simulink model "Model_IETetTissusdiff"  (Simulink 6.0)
settings: Solver=ode45  StartTime=0.0  StopTime=16*t0  RelTol=1e-3
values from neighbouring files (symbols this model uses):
  beta = 0.95    [Constantes.m]    (also in ConstantesBck.m; ResCourV1.m = 1; ResCrV1.m = 1; ResEnerV1.m = 1)
  C = 1    [Constantes.m]    (also in ConstantesBck.m)
  Cdl = 603E-9    (= 6.03e-07)    [Constantes.m]    (also in ConstantesBck.m; ResCourV1.m = 7.313e-07; ResCrV1.m = 7.313e-07; ResEnerV1.m = 7.313e-07)
  const = 1E4    (= 10000)    [ConstantesBck.m]
  Fact = 10^2    (= 100)    [Constantes.m]    (also in ConstantesBck.m)
  gk = 36    [Constantes.m]    (also in ConstantesBck.m; sim_hh.m)
  gl = 0.3    [Constantes.m]    (also in ConstantesBck.m; sim_hh.m)
  gna = 120    [Constantes.m]    (also in ConstantesBck.m; sim_hh.m)
  h0 = 0.5961    [Constantes.m]    (also in ConstantesBck.m)
  Istim = 200E-6    (= 0.0002)    [Constantes.m]    (also in ConstantesBck.m = 5e-05)
  k = vth/pot    [CalculCharge.m]
  m0 = 0.0529    [Constantes.m]    (also in ConstantesBck.m)
  n0 = 0.3177    [Constantes.m]    (also in ConstantesBck.m)
  Rct = 185.6E3    (= 185600)    [Constantes.m]    (also in ConstantesBck.m; ResCourV1.m = 605200; ResCrV1.m = 605200; ResEnerV1.m = 605200)
  Rext = 2.9E3    (= 2900)    [Constantes.m]    (also in ConstantesBck.m)
  Rint = 2.9E2    (= 290)    [Constantes.m]    (also in ConstantesBck.m = 400)
  S = 3.14E-3    (= 0.00314)    [Constantes.m]    (also in ConstantesBck.m = 3.14e-09; ImpedanceZtissus.m = 4e-06; Ztissus.m = 4e-06)
  sigma = 66466    [Constantes.m]    (also in ConstantesBck.m; ResCourV1.m = 68000; ResCrV1.m = 68000; ResEnerV1.m = 68000)
  t0 = 2E-3    (= 0.002)    [Constantes.m]    (also in ConstantesBck.m = 0.001)
  Vdd = 3.3*Rcan/Rct*1000    (= 3.2147881681)    [Constantes.m]    (also in ConstantesBck.m = 1.8)
  Vk = -82    [Constantes.m]    (also in ConstantesBck.m)
  Vl = -59    [Constantes.m]    (also in ConstantesBck.m)
  Vna = 45    [Constantes.m]    (also in ConstantesBck.m)

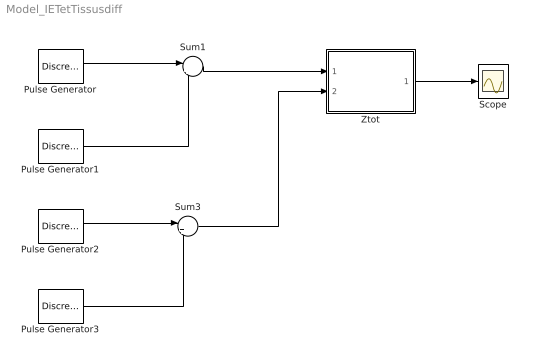
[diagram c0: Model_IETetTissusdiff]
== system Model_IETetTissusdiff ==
  Pulse Generator : DiscretePulseGenerator  PulseType=Time based  Amplitude=-Istim  Period=t0  PulseWidth=50
  Pulse Generator1 : DiscretePulseGenerator  PulseType=Time based  Amplitude=Istim  Period=t0  PulseWidth=50  PhaseDelay=t0/2
  Pulse Generator2 : DiscretePulseGenerator  PulseType=Time based  Amplitude=Vdd/2  Period=t0  PulseWidth=50
  Pulse Generator3 : DiscretePulseGenerator  PulseType=Time based  Amplitude=-Vdd/2  Period=t0  PulseWidth=50  PhaseDelay=t0/2
  Scope : Scope
  Sum1 : Sum  Inputs=|++
  Sum3 : Sum  Inputs=|++
  Ztot : Subsystem
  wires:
  Pulse Generator/1 -> Sum1/1
  Pulse Generator1/1 -> Sum1/2
  Sum1/1 -> Ztot/1(InZtot)
  Pulse Generator2/1 -> Sum3/1
  Pulse Generator3/1 -> Sum3/2
  Ztot/1(OutZtot) -> Scope/1
  Sum3/1 -> Ztot/2(InVRef)

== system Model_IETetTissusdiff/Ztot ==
  InZtot : Inport  Port=1  LatchInput=off
  InVRef : Inport  Port=2  LatchInput=off
  Gain : Gain
  Sum : Sum  Inputs=|++
  ZTissus : Subsystem
  Ziet : Subsystem
  OutZtot : Outport
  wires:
  Ziet/1(OutZiet) -> Gain/1
  InZtot/1 -> Ziet/1(InZiet), ZTissus/1(IStim)
  Gain/1 -> Sum/2
  Sum/1 -> OutZtot/1
  InVRef/1 -> ZTissus/2(Vref)
  ZTissus/1(Vout) -> Sum/1

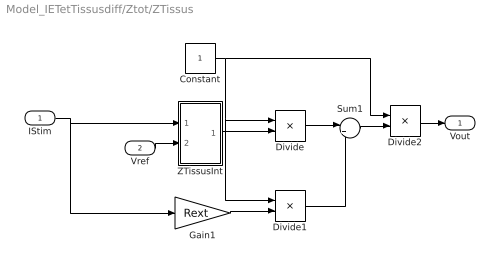
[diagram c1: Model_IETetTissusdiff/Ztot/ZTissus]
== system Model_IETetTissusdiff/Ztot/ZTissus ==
  IStim : Inport  Port=1  LatchInput=off
  Vref : Inport  Port=2  LatchInput=off
  Constant : Constant
  Divide : Product  Inputs=*/  OutScaling=2^-10
  Divide1 : Product  Inputs=*/  OutScaling=2^-10
  Divide2 : Product  Inputs=*/  OutScaling=2^-10
  Gain1 : Gain  Gain=Rext
  Sum1 : Sum  Inputs=|++
  ZTissusInt : Subsystem
  Vout : Outport
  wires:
  IStim/1 -> ZTissusInt/1(InStim), Gain1/1
  Constant/1 -> Divide/1, Divide1/1, Divide2/1
  ZTissusInt/1(Vout) -> Divide/2
  Gain1/1 -> Divide1/2
  Divide/1 -> Sum1/1
  Divide1/1 -> Sum1/2
  Sum1/1 -> Divide2/2
  Divide2/1 -> Vout/1
  Vref/1 -> ZTissusInt/2(VRefIn)

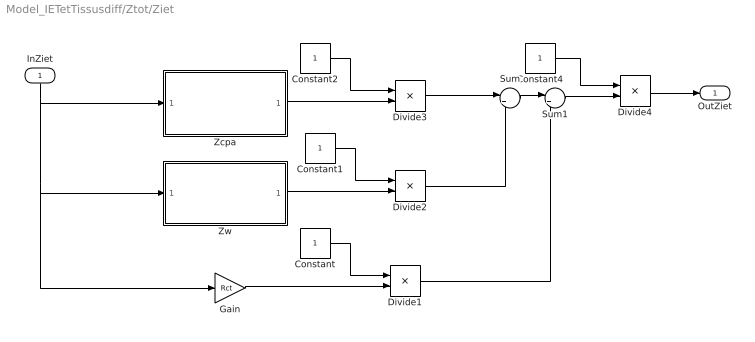
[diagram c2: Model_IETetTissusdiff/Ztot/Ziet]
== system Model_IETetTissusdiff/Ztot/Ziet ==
  InZiet : Inport  Orientation=down  Port=1  LatchInput=off
  Constant{,1..2,4} (4 alike) : Constant
  Divide{1..4} (4 alike) : Product  Inputs=*/  OutScaling=2^-10
  Gain : Gain  Gain=Rct
  Sum : Sum  Inputs=|++
  Sum1 : Sum  Inputs=|++
  Zcpa : Subsystem
  Zw : Subsystem
  OutZiet : Outport
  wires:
  Constant/1 -> Divide1/1
  Constant1/1 -> Divide2/1
  Constant2/1 -> Divide3/1
  Zcpa/1(OutZcpa) -> Divide3/2
  Zw/1(OutZw) -> Divide2/2
  Gain/1 -> Divide1/2
  Divide3/1 -> Sum/1
  Constant4/1 -> Divide4/1
  InZiet/1 -> Zcpa/1(InZcpa), Zw/1(InZw), Gain/1
  Divide4/1 -> OutZiet/1
  Divide2/1 -> Sum/2
  Sum/1 -> Sum1/1
  Divide1/1 -> Sum1/2
  Sum1/1 -> Divide4/2

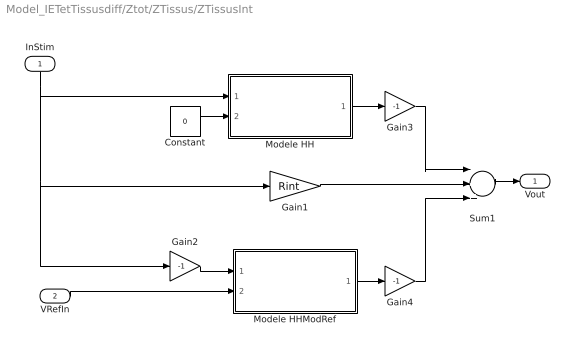
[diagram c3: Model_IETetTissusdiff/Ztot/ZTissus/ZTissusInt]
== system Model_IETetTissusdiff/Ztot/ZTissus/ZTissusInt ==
  InStim : Inport  Orientation=down  Port=1  LatchInput=off
  VRefIn : Inport  Port=2  LatchInput=off
  Constant : Constant  Value=0
  Gain1 : Gain  Gain=Rint
  Gain2 : Gain  Gain=-1
  Gain3 : Gain  Gain=-1
  Gain4 : Gain  Gain=-1
  Modele HH : Subsystem
  Modele HHModRef : Subsystem
  Sum1 : Sum  Inputs=|+++
  Vout : Outport
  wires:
  Modele HH/1(HHout) -> Gain3/1
  Modele HHModRef/1(HHout) -> Gain4/1
  Gain1/1 -> Sum1/2
  Gain2/1 -> Modele HHModRef/1(HHin)
  InStim/1 -> Gain1/1, Gain2/1, Modele HH/1(HHin)
  Constant/1 -> Modele HH/2(VRefIn)
  Sum1/1 -> Vout/1
  VRefIn/1 -> Modele HHModRef/2(VRefIn)
  Gain3/1 -> Sum1/1
  Gain4/1 -> Sum1/3

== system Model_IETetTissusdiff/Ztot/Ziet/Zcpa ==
  InZcpa : Inport  Port=1  LatchInput=off
  Fcn : Fcn  Expr=u(1)^beta
  Transfer Fcn : TransferFcn  Denominator=[Cdl 0]
  OutZcpa : Outport
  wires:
  Transfer Fcn/1 -> Fcn/1
  InZcpa/1 -> Transfer Fcn/1
  Fcn/1 -> OutZcpa/1

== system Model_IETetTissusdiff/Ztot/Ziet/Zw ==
  InZw : Inport  Port=1  LatchInput=off
  Gain : Gain  Gain=sigma
  Math Function : Math  Operator=sqrt
  Transfer Fcn : TransferFcn  Numerator=[2]  Denominator=[1 0]
  OutZw : Outport
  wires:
  Transfer Fcn/1 -> Math Function/1
  Math Function/1 -> Gain/1
  Gain/1 -> OutZw/1
  InZw/1 -> Transfer Fcn/1

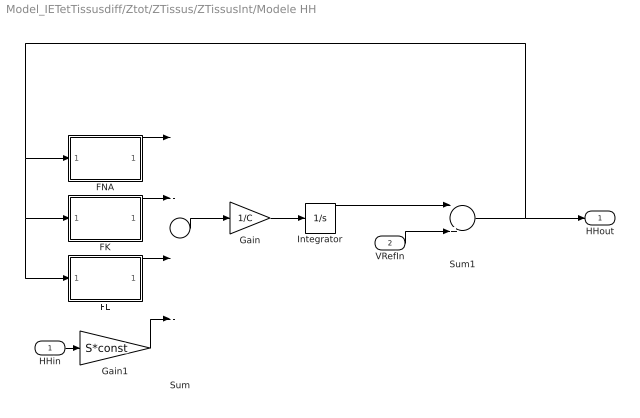
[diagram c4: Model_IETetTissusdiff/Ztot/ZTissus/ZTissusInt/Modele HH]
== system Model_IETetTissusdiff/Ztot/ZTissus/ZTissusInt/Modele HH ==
  HHin : Inport  Port=1  LatchInput=off
  VRefIn : Inport  Port=2  LatchInput=off
  FK : Subsystem
  FL : Subsystem
  FNA : Subsystem
  Gain : Gain  Gain=1/C
  Gain1 : Gain  Gain=S*const
  Integrator : Integrator
  Sum : Sum  Inputs=|---+
  Sum1 : Sum  Inputs=|++
  HHout : Outport
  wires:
  Sum/1 -> Gain/1
  Gain/1 -> Integrator/1
  FNA/1(FNAout) -> Sum/1
  FK/1(FKout) -> Sum/2
  FL/1(FLout) -> Sum/3
  HHin/1 -> Gain1/1
  Integrator/1 -> Sum1/1
  Sum1/1 -> HHout/1, FNA/1(FNAin), FK/1(FKin), FL/1(FLin)
  VRefIn/1 -> Sum1/2
  Gain1/1 -> Sum/4

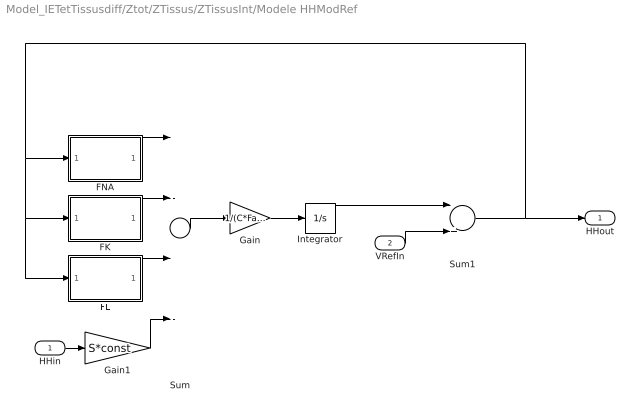
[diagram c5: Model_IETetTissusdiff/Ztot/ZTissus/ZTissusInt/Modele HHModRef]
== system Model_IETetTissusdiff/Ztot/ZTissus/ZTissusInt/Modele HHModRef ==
  HHin : Inport  Port=1  LatchInput=off
  VRefIn : Inport  Port=2  LatchInput=off
  FK : Subsystem
  FL : Subsystem
  FNA : Subsystem
  Gain : Gain  Gain=1/(C*Fact)
  Gain1 : Gain  Gain=S*const
  Integrator : Integrator
  Sum : Sum  Inputs=|---+
  Sum1 : Sum  Inputs=|++
  HHout : Outport
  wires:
  Sum/1 -> Gain/1
  Gain/1 -> Integrator/1
  FNA/1(FNAout) -> Sum/1
  FK/1(FKout) -> Sum/2
  FL/1(FLout) -> Sum/3
  HHin/1 -> Gain1/1
  Integrator/1 -> Sum1/1
  Sum1/1 -> HHout/1, FNA/1(FNAin), FK/1(FKin), FL/1(FLin)
  VRefIn/1 -> Sum1/2
  Gain1/1 -> Sum/4

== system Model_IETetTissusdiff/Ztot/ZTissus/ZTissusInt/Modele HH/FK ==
  FKin : Inport  Orientation=down  Port=1  LatchInput=off
  Constant1 : Constant  Value=Vk
  Fcn : Fcn  Expr=u^4
  Gain : Gain  Gain=-gk
  Product : Product
  Sum1 : Sum  Inputs=|+-
  n(t) : Subsystem
  FKout : Outport
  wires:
  n(t)/1(nout) -> Fcn/1
  Constant1/1 -> Sum1/2
  FKin/1 -> n(t)/1(nin), Sum1/1
  Product/1 -> Gain/1
  Fcn/1 -> Product/1
  Sum1/1 -> Product/2
  Gain/1 -> FKout/1

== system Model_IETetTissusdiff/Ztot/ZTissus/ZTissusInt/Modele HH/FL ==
  FLin : Inport  Orientation=down  Port=1  LatchInput=off
  Constant1 : Constant  Value=Vl
  Gain : Gain  Gain=-gl
  Sum1 : Sum  Inputs=|+-
  FLout : Outport
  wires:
  Constant1/1 -> Sum1/2
  FLin/1 -> Sum1/1
  Sum1/1 -> Gain/1
  Gain/1 -> FLout/1

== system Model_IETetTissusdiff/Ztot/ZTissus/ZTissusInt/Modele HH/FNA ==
  FNAin : Inport  Port=1  LatchInput=off
  Constant : Constant  Value=Vna
  Fcn : Fcn  Expr=u^3
  Gain : Gain  Gain=-gna
  Product : Product  Inputs=3
  Sum1 : Sum  Inputs=|+-
  h(t) : Subsystem
  m(t) : Subsystem
  FNAout : Outport
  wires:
  Sum1/1 -> Product/1
  Constant/1 -> Sum1/2
  FNAin/1 -> h(t)/1(hin), m(t)/1(min), Sum1/1
  m(t)/1(mout) -> Fcn/1
  Product/1 -> Gain/1
  Fcn/1 -> Product/2
  h(t)/1(hout) -> Product/3
  Gain/1 -> FNAout/1

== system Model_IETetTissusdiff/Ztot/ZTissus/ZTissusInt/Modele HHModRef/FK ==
  FKin : Inport  Orientation=down  Port=1  LatchInput=off
  Constant1 : Constant  Value=Vk
  Fcn : Fcn  Expr=u^4
  Gain : Gain  Gain=-gk*Fact
  Product : Product
  Sum1 : Sum  Inputs=|+-
  n(t) : Subsystem
  FKout : Outport
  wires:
  n(t)/1(nout) -> Fcn/1
  Constant1/1 -> Sum1/2
  FKin/1 -> n(t)/1(nin), Sum1/1
  Product/1 -> Gain/1
  Fcn/1 -> Product/1
  Sum1/1 -> Product/2
  Gain/1 -> FKout/1

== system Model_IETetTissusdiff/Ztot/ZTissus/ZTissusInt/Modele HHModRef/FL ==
  FLin : Inport  Orientation=down  Port=1  LatchInput=off
  Constant1 : Constant  Value=Vl
  Gain : Gain  Gain=-gl*Fact
  Sum1 : Sum  Inputs=|+-
  FLout : Outport
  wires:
  Constant1/1 -> Sum1/2
  FLin/1 -> Sum1/1
  Sum1/1 -> Gain/1
  Gain/1 -> FLout/1

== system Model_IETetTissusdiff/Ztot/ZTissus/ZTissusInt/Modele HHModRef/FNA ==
  FNAin : Inport  Port=1  LatchInput=off
  Constant : Constant  Value=Vna
  Fcn : Fcn  Expr=u^3
  Gain : Gain  Gain=-gna*Fact
  Product : Product  Inputs=3
  Sum1 : Sum  Inputs=|+-
  h(t) : Subsystem
  m(t) : Subsystem
  FNAout : Outport
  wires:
  Sum1/1 -> Product/1
  Constant/1 -> Sum1/2
  FNAin/1 -> h(t)/1(hin), m(t)/1(min), Sum1/1
  m(t)/1(mout) -> Fcn/1
  Product/1 -> Gain/1
  Fcn/1 -> Product/2
  h(t)/1(hout) -> Product/3
  Gain/1 -> FNAout/1

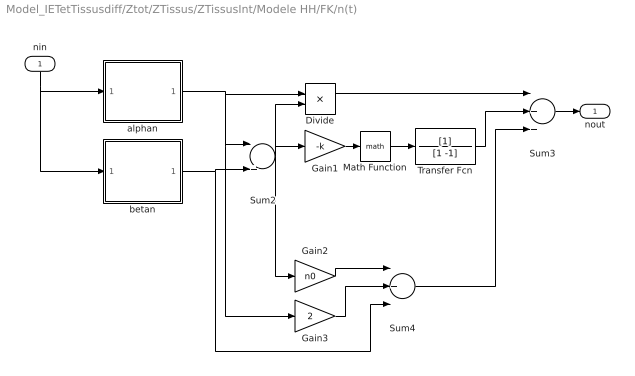
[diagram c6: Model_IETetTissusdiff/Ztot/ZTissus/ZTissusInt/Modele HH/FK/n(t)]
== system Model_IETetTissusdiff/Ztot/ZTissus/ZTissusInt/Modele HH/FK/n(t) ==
  nin : Inport  Orientation=down  Port=1  LatchInput=off
  Divide : Product  Inputs=*/  OutScaling=2^-10
  Gain1 : Gain  Gain=-k
  Gain2 : Gain  Gain=n0
  Gain3 : Gain  Gain=2
  Math Function : Math
  Sum2 : Sum  Inputs=|++
  Sum3 : Sum  Inputs=|+++
  Sum4 : Sum  Inputs=|+--
  Transfer Fcn : TransferFcn  Denominator=[1 -1]
  alphan : Subsystem
  betan : Subsystem
  nout : Outport
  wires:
  Divide/1 -> Sum3/1
  Sum2/1 -> Gain1/1, Divide/2, Gain2/1
  Gain1/1 -> Math Function/1
  Math Function/1 -> Transfer Fcn/1
  Gain2/1 -> Sum4/1
  Gain3/1 -> Sum4/2
  Sum4/1 -> Sum3/3
  nin/1 -> alphan/1(anin), betan/1(bnin)
  Sum3/1 -> nout/1
  alphan/1(anout) -> Divide/1, Sum2/1, Gain3/1
  betan/1(bnout) -> Sum2/2, Sum4/3
  Transfer Fcn/1 -> Sum3/2

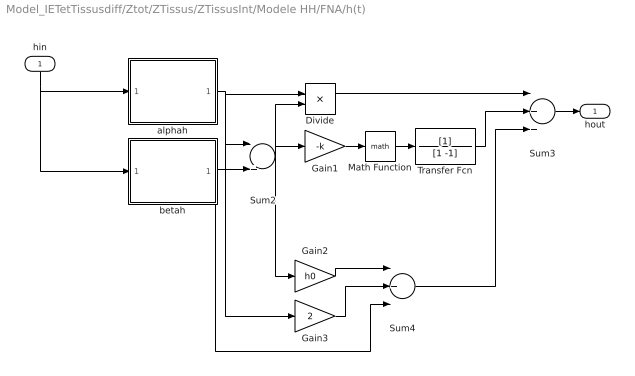
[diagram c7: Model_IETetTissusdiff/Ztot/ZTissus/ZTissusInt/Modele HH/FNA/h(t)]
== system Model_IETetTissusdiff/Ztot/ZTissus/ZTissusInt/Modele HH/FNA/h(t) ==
  hin : Inport  Orientation=down  Port=1  LatchInput=off
  Divide : Product  Inputs=*/  OutScaling=2^-10
  Gain1 : Gain  Gain=-k
  Gain2 : Gain  Gain=h0
  Gain3 : Gain  Gain=2
  Math Function : Math
  Sum2 : Sum  Inputs=|++
  Sum3 : Sum  Inputs=|+++
  Sum4 : Sum  Inputs=|+--
  Transfer Fcn : TransferFcn  Denominator=[1 -1]
  alphah : Subsystem
  betah : Subsystem
  hout : Outport
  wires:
  alphah/1(ahout) -> Divide/1, Sum2/1, Gain3/1
  betah/1(bhout) -> Sum2/2, Sum4/3
  Divide/1 -> Sum3/1
  Sum2/1 -> Gain1/1, Divide/2, Gain2/1
  Gain1/1 -> Math Function/1
  Math Function/1 -> Transfer Fcn/1
  Gain2/1 -> Sum4/1
  Gain3/1 -> Sum4/2
  Sum4/1 -> Sum3/3
  hin/1 -> betah/1(bhin), alphah/1(ahin)
  Sum3/1 -> hout/1
  Transfer Fcn/1 -> Sum3/2

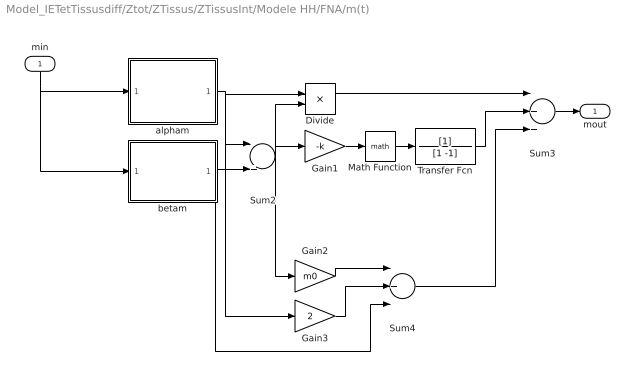
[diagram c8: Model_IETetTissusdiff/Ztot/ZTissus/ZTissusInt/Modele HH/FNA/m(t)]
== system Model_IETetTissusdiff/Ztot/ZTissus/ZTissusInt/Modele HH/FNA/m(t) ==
  min : Inport  Orientation=down  Port=1  LatchInput=off
  Divide : Product  Inputs=*/  OutScaling=2^-10
  Gain1 : Gain  Gain=-k
  Gain2 : Gain  Gain=m0
  Gain3 : Gain  Gain=2
  Math Function : Math
  Sum2 : Sum  Inputs=|++
  Sum3 : Sum  Inputs=|+++
  Sum4 : Sum  Inputs=|+--
  Transfer Fcn : TransferFcn  Denominator=[1 -1]
  alpham : Subsystem
  betam : Subsystem
  mout : Outport
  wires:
  alpham/1(amout) -> Divide/1, Sum2/1, Gain3/1
  betam/1(bmout) -> Sum2/2, Sum4/3
  Divide/1 -> Sum3/1
  Sum2/1 -> Gain1/1, Divide/2, Gain2/1
  Gain1/1 -> Math Function/1
  Math Function/1 -> Transfer Fcn/1
  Gain2/1 -> Sum4/1
  Gain3/1 -> Sum4/2
  Sum4/1 -> Sum3/3
  min/1 -> alpham/1(amin), betam/1(bmin)
  Sum3/1 -> mout/1
  Transfer Fcn/1 -> Sum3/2

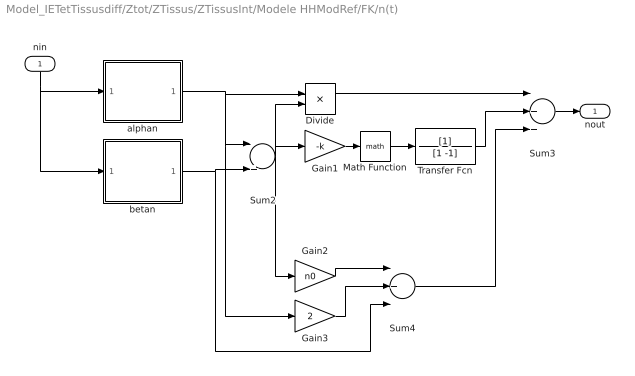
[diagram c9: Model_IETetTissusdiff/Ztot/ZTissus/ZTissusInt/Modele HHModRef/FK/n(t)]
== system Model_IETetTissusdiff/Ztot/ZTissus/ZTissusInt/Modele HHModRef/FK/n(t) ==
  nin : Inport  Orientation=down  Port=1  LatchInput=off
  Divide : Product  Inputs=*/  OutScaling=2^-10
  Gain1 : Gain  Gain=-k
  Gain2 : Gain  Gain=n0
  Gain3 : Gain  Gain=2
  Math Function : Math
  Sum2 : Sum  Inputs=|++
  Sum3 : Sum  Inputs=|+++
  Sum4 : Sum  Inputs=|+--
  Transfer Fcn : TransferFcn  Denominator=[1 -1]
  alphan : Subsystem
  betan : Subsystem
  nout : Outport
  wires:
  Divide/1 -> Sum3/1
  Sum2/1 -> Gain1/1, Divide/2, Gain2/1
  Gain1/1 -> Math Function/1
  Math Function/1 -> Transfer Fcn/1
  Gain2/1 -> Sum4/1
  Gain3/1 -> Sum4/2
  Sum4/1 -> Sum3/3
  nin/1 -> alphan/1(anin), betan/1(bnin)
  Sum3/1 -> nout/1
  alphan/1(anout) -> Divide/1, Sum2/1, Gain3/1
  betan/1(bnout) -> Sum2/2, Sum4/3
  Transfer Fcn/1 -> Sum3/2

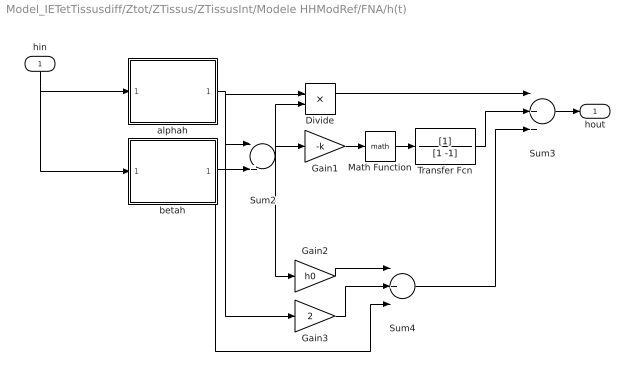
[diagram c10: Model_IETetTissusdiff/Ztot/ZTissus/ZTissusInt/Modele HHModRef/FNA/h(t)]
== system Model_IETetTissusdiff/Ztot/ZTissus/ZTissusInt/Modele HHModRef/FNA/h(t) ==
  hin : Inport  Orientation=down  Port=1  LatchInput=off
  Divide : Product  Inputs=*/  OutScaling=2^-10
  Gain1 : Gain  Gain=-k
  Gain2 : Gain  Gain=h0
  Gain3 : Gain  Gain=2
  Math Function : Math
  Sum2 : Sum  Inputs=|++
  Sum3 : Sum  Inputs=|+++
  Sum4 : Sum  Inputs=|+--
  Transfer Fcn : TransferFcn  Denominator=[1 -1]
  alphah : Subsystem
  betah : Subsystem
  hout : Outport
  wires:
  alphah/1(ahout) -> Divide/1, Sum2/1, Gain3/1
  betah/1(bhout) -> Sum2/2, Sum4/3
  Divide/1 -> Sum3/1
  Sum2/1 -> Gain1/1, Divide/2, Gain2/1
  Gain1/1 -> Math Function/1
  Math Function/1 -> Transfer Fcn/1
  Gain2/1 -> Sum4/1
  Gain3/1 -> Sum4/2
  Sum4/1 -> Sum3/3
  hin/1 -> betah/1(bhin), alphah/1(ahin)
  Sum3/1 -> hout/1
  Transfer Fcn/1 -> Sum3/2

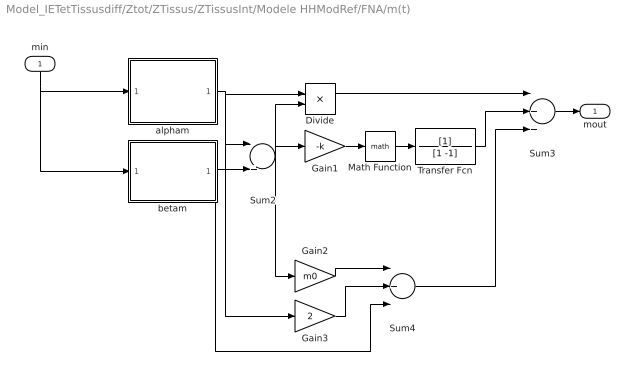
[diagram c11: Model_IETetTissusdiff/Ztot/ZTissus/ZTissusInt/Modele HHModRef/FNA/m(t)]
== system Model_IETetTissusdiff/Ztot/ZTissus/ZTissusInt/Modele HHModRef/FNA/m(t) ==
  min : Inport  Orientation=down  Port=1  LatchInput=off
  Divide : Product  Inputs=*/  OutScaling=2^-10
  Gain1 : Gain  Gain=-k
  Gain2 : Gain  Gain=m0
  Gain3 : Gain  Gain=2
  Math Function : Math
  Sum2 : Sum  Inputs=|++
  Sum3 : Sum  Inputs=|+++
  Sum4 : Sum  Inputs=|+--
  Transfer Fcn : TransferFcn  Denominator=[1 -1]
  alpham : Subsystem
  betam : Subsystem
  mout : Outport
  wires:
  alpham/1(amout) -> Divide/1, Sum2/1, Gain3/1
  betam/1(bmout) -> Sum2/2, Sum4/3
  Divide/1 -> Sum3/1
  Sum2/1 -> Gain1/1, Divide/2, Gain2/1
  Gain1/1 -> Math Function/1
  Math Function/1 -> Transfer Fcn/1
  Gain2/1 -> Sum4/1
  Gain3/1 -> Sum4/2
  Sum4/1 -> Sum3/3
  min/1 -> alpham/1(amin), betam/1(bmin)
  Sum3/1 -> mout/1
  Transfer Fcn/1 -> Sum3/2

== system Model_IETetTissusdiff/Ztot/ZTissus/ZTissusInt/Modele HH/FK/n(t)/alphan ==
  anin : Inport  Port=1  LatchInput=off
  Constant : Constant
  Divide1 : Product  Inputs=*/  OutScaling=2^-10
  Gain4 : Gain  Gain=0.1
  Gain5 : Gain  Gain=1/10
  Math Function1 : Math
  Sum : Sum  Inputs=|+-
  Sum1 : Sum  Inputs=|+-
  anout : Outport
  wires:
  Sum1/1 -> Divide1/2
  Gain5/1 -> Divide1/1
  Math Function1/1 -> Sum1/1
  Sum/1 -> Math Function1/1, Gain5/1
  Gain4/1 -> Sum/2
  Constant/1 -> Sum/1, Sum1/2
  anin/1 -> Gain4/1
  Divide1/1 -> anout/1

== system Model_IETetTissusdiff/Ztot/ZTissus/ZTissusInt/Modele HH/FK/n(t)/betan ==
  bnin : Inport  Port=1  LatchInput=off
  Gain4 : Gain  Gain=-1/80
  Gain5 : Gain  Gain=0.125
  Math Function1 : Math
  bnout : Outport
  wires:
  Gain4/1 -> Math Function1/1
  Math Function1/1 -> Gain5/1
  bnin/1 -> Gain4/1
  Gain5/1 -> bnout/1

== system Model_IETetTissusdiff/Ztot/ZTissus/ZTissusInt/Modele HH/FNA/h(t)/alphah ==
  ahin : Inport  Port=1  LatchInput=off
  Gain4 : Gain  Gain=-1/20
  Gain5 : Gain  Gain=0.07
  Math Function1 : Math
  ahout : Outport
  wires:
  Gain4/1 -> Math Function1/1
  Math Function1/1 -> Gain5/1
  ahin/1 -> Gain4/1
  Gain5/1 -> ahout/1

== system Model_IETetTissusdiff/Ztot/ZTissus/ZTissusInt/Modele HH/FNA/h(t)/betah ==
  bhin : Inport  Port=1  LatchInput=off
  Add : Sum  Inputs=+-  OutScaling=2^-10
  Add1 : Sum  OutScaling=2^-10
  Constant3 : Constant
  Constant4 : Constant  Value=3
  Divide1 : Product  Inputs=*/  OutScaling=2^-10
  Gain4 : Gain  Gain=0.1
  Math Function1 : Math
  bhout : Outport
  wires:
  Constant3/1 -> Divide1/1, Add1/1
  Constant4/1 -> Add/1
  Gain4/1 -> Add/2
  Add/1 -> Math Function1/1
  Math Function1/1 -> Add1/2
  Add1/1 -> Divide1/2
  bhin/1 -> Gain4/1
  Divide1/1 -> bhout/1

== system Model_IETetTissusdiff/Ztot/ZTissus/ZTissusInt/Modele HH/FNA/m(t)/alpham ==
  amin : Inport  Port=1  LatchInput=off
  Constant2 : Constant  Value=2.5
  Constant3 : Constant
  Divide : Product  Inputs=*/  OutScaling=2^-10
  Gain1 : Gain  Gain=0.1
  Math Function : Math
  Sum2 : Sum  Inputs=|++
  Sum3 : Sum  Inputs=|++
  amout : Outport
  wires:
  Constant2/1 -> Sum2/1
  Gain1/1 -> Sum2/2
  Sum2/1 -> Divide/1, Math Function/1
  Sum3/1 -> Divide/2
  Constant3/1 -> Sum3/2
  Math Function/1 -> Sum3/1
  amin/1 -> Gain1/1
  Divide/1 -> amout/1

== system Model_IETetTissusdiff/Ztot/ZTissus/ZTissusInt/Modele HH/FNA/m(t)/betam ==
  bmin : Inport  Port=1  LatchInput=off
  Gain1 : Gain  Gain=-1/18
  Gain2 : Gain  Gain=4
  Math Function : Math
  bmout : Outport
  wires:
  Gain1/1 -> Math Function/1
  Math Function/1 -> Gain2/1
  bmin/1 -> Gain1/1
  Gain2/1 -> bmout/1

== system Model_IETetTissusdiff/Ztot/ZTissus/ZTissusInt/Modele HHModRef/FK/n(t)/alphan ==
  anin : Inport  Port=1  LatchInput=off
  Constant : Constant
  Divide1 : Product  Inputs=*/  OutScaling=2^-10
  Gain4 : Gain  Gain=0.1
  Gain5 : Gain  Gain=1/10
  Math Function1 : Math
  Sum : Sum  Inputs=|+-
  Sum1 : Sum  Inputs=|+-
  anout : Outport
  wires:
  Sum1/1 -> Divide1/2
  Gain5/1 -> Divide1/1
  Math Function1/1 -> Sum1/1
  Sum/1 -> Math Function1/1, Gain5/1
  Gain4/1 -> Sum/2
  Constant/1 -> Sum/1, Sum1/2
  anin/1 -> Gain4/1
  Divide1/1 -> anout/1

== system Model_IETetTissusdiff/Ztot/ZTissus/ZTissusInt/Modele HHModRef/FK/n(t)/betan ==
  bnin : Inport  Port=1  LatchInput=off
  Gain4 : Gain  Gain=-1/80
  Gain5 : Gain  Gain=0.125
  Math Function1 : Math
  bnout : Outport
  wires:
  Gain4/1 -> Math Function1/1
  Math Function1/1 -> Gain5/1
  bnin/1 -> Gain4/1
  Gain5/1 -> bnout/1

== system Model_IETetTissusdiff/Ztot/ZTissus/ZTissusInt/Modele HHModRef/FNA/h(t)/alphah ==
  ahin : Inport  Port=1  LatchInput=off
  Gain4 : Gain  Gain=-1/20
  Gain5 : Gain  Gain=0.07
  Math Function1 : Math
  ahout : Outport
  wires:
  Gain4/1 -> Math Function1/1
  Math Function1/1 -> Gain5/1
  ahin/1 -> Gain4/1
  Gain5/1 -> ahout/1

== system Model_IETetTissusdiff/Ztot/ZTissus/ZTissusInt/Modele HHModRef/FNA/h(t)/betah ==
  bhin : Inport  Port=1  LatchInput=off
  Add : Sum  Inputs=+-  OutScaling=2^-10
  Add1 : Sum  OutScaling=2^-10
  Constant3 : Constant
  Constant4 : Constant  Value=3
  Divide1 : Product  Inputs=*/  OutScaling=2^-10
  Gain4 : Gain  Gain=0.1
  Math Function1 : Math
  bhout : Outport
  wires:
  Constant3/1 -> Divide1/1, Add1/1
  Constant4/1 -> Add/1
  Gain4/1 -> Add/2
  Add/1 -> Math Function1/1
  Math Function1/1 -> Add1/2
  Add1/1 -> Divide1/2
  bhin/1 -> Gain4/1
  Divide1/1 -> bhout/1

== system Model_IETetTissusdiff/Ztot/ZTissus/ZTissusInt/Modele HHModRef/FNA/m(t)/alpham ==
  amin : Inport  Port=1  LatchInput=off
  Constant2 : Constant  Value=2.5
  Constant3 : Constant
  Divide : Product  Inputs=*/  OutScaling=2^-10
  Gain1 : Gain  Gain=0.1
  Math Function : Math
  Sum2 : Sum  Inputs=|++
  Sum3 : Sum  Inputs=|++
  amout : Outport
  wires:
  Constant2/1 -> Sum2/1
  Gain1/1 -> Sum2/2
  Sum2/1 -> Divide/1, Math Function/1
  Sum3/1 -> Divide/2
  Constant3/1 -> Sum3/2
  Math Function/1 -> Sum3/1
  amin/1 -> Gain1/1
  Divide/1 -> amout/1

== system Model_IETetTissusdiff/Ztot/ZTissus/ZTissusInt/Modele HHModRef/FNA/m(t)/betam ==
  bmin : Inport  Port=1  LatchInput=off
  Gain1 : Gain  Gain=-1/18
  Gain2 : Gain  Gain=4
  Math Function : Math
  bmout : Outport
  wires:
  Gain1/1 -> Math Function/1
  Math Function/1 -> Gain2/1
  bmin/1 -> Gain1/1
  Gain2/1 -> bmout/1
